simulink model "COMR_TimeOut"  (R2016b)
settings: Solver=FixedStepDiscrete  StartTime=0.0  StopTime=10.0  FixedStep=0.01  RelTol=1e-3  EnableMultiTasking=on
undefined symbols (not defined in the file or in its folder): bin2dec, COMR_cntObcTmtDiag_CW, COMR_cntVcu2A3TmtDiag_CW, COMR_flgTmtCAB_C, COMR_numPackVcuMsg_C, COMR_tiBusoffDiagEna_C, COMR_tiCabMsgTmt_C, COMR_tiCSCMsgTmt_C, COMR_tiGWMsg050Tmt_C, COMR_tiGWMsgTmt_C, COMR_tiHv638MsgTmt_C, COMR_tiMcuMsgTmt_C, COMR_tiObcMsgTmt_C, COMR_tiPackVcuMsgTmt_C, COMR_tiPwrupDiagEna_C, COMR_tiTmtBase_C, COMR_tiVcuMsgTmt_C, COMR_UAESFltDiagDisbl_C
libraries: simulink x167
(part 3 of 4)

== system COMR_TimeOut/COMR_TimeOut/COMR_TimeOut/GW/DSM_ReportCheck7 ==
  note: Fault report to diagnostic management system
  Dfc_id_nv : Inport  OutDataTypeStr=uint8
  Err : Inport  Port=2
  Heal : Inport  Port=3
  Bit Clear1 : simulink/Logic and Bit Operations/Bit Clear  iBit=4
  Bit Clear2 : simulink/Logic and Bit Operations/Bit Clear  iBit=3
  Bit Set : simulink/Logic and Bit Operations/Bit Set  iBit=4
  Bit Set1 : simulink/Logic and Bit Operations/Bit Set  iBit=3
  Bit Set2 : simulink/Logic and Bit Operations/Bit Set  iBit=3
  Bit Set4 : simulink/Logic and Bit Operations/Bit Set  iBit=7
  Constant1 : Constant  Value=0  OutDataTypeStr=uint8
  Constant7 : Constant  Value=0  OutDataTypeStr=boolean
  Delay2 : Delay  DelayLength=1  InitialCondition=1
  Delay3 : Delay  DelayLength=1  InitialCondition=0
  Logical Operator : Logic  Operator=OR  AllPortsSameDT=off  OutDataTypeStr=boolean
  Switch{1..4} (4 alike) : Switch  Criteria=u2 ~= 0
  Dfc_id : Outport  OutDataTypeStr=uint8
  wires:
  Switch1/1 -> Dfc_id/1
  Constant1/1 -> Switch1/3
  Logical Operator/1 -> Switch1/2
  Heal/1 -> Switch4/2, Logical Operator/1
  Delay3/1 -> Switch4/3
  Bit Clear1/1 -> Bit Set2/1
  Bit Set2/1 -> Switch4/1
  Err/1 -> Switch3/2, Logical Operator/2
  Switch4/1 -> Switch3/3
  Bit Set/1 -> Bit Set1/1
  Bit Set1/1 -> Switch3/1
  Switch2/1 -> Switch1/1, Delay3/1
  Bit Clear2/1 -> Switch2/1
  Switch3/1 -> Switch2/3
  Delay2/1 -> Switch2/2
  Constant7/1 -> Delay2/1
  Bit Set4/1 -> Bit Set/1
  Dfc_id_nv/1 -> Bit Clear1/1, Bit Set4/1, Bit Clear2/1

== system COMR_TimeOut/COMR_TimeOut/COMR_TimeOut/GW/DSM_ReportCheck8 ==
  note: Fault report to diagnostic management system
  Dfc_id_nv : Inport  OutDataTypeStr=uint8
  Err : Inport  Port=2
  Heal : Inport  Port=3
  Bit Clear1 : simulink/Logic and Bit Operations/Bit Clear  iBit=4
  Bit Clear2 : simulink/Logic and Bit Operations/Bit Clear  iBit=3
  Bit Set : simulink/Logic and Bit Operations/Bit Set  iBit=4
  Bit Set1 : simulink/Logic and Bit Operations/Bit Set  iBit=3
  Bit Set2 : simulink/Logic and Bit Operations/Bit Set  iBit=3
  Bit Set4 : simulink/Logic and Bit Operations/Bit Set  iBit=7
  Constant1 : Constant  Value=0  OutDataTypeStr=uint8
  Constant7 : Constant  Value=0  OutDataTypeStr=boolean
  Delay2 : Delay  DelayLength=1  InitialCondition=1
  Delay3 : Delay  DelayLength=1  InitialCondition=0
  Logical Operator : Logic  Operator=OR  AllPortsSameDT=off  OutDataTypeStr=boolean
  Switch{1..4} (4 alike) : Switch  Criteria=u2 ~= 0
  Dfc_id : Outport  OutDataTypeStr=uint8
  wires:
  Dfc_id_nv/1 -> Bit Clear2/1, Bit Set4/1, Bit Clear1/1
  Bit Set4/1 -> Bit Set/1
  Constant7/1 -> Delay2/1
  Delay2/1 -> Switch2/2
  Switch3/1 -> Switch2/3
  Bit Clear2/1 -> Switch2/1
  Switch2/1 -> Delay3/1, Switch1/1
  Bit Set1/1 -> Switch3/1
  Bit Set/1 -> Bit Set1/1
  Switch4/1 -> Switch3/3
  Err/1 -> Logical Operator/2, Switch3/2
  Bit Set2/1 -> Switch4/1
  Bit Clear1/1 -> Bit Set2/1
  Delay3/1 -> Switch4/3
  Heal/1 -> Logical Operator/1, Switch4/2
  Logical Operator/1 -> Switch1/2
  Constant1/1 -> Switch1/3
  Switch1/1 -> Dfc_id/1

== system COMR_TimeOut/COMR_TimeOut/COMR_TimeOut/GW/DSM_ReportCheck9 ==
  note: Fault report to diagnostic management system
  Dfc_id_nv : Inport  OutDataTypeStr=uint8
  Err : Inport  Port=2
  Heal : Inport  Port=3
  Bit Clear1 : simulink/Logic and Bit Operations/Bit Clear  iBit=4
  Bit Clear2 : simulink/Logic and Bit Operations/Bit Clear  iBit=3
  Bit Set : simulink/Logic and Bit Operations/Bit Set  iBit=4
  Bit Set1 : simulink/Logic and Bit Operations/Bit Set  iBit=3
  Bit Set2 : simulink/Logic and Bit Operations/Bit Set  iBit=3
  Bit Set4 : simulink/Logic and Bit Operations/Bit Set  iBit=7
  Constant1 : Constant  Value=0  OutDataTypeStr=uint8
  Constant7 : Constant  Value=0  OutDataTypeStr=boolean
  Delay2 : Delay  DelayLength=1  InitialCondition=1
  Delay3 : Delay  DelayLength=1  InitialCondition=0
  Logical Operator : Logic  Operator=OR  AllPortsSameDT=off  OutDataTypeStr=boolean
  Switch{1..4} (4 alike) : Switch  Criteria=u2 ~= 0
  Dfc_id : Outport  OutDataTypeStr=uint8
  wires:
  Switch1/1 -> Dfc_id/1
  Constant1/1 -> Switch1/3
  Logical Operator/1 -> Switch1/2
  Heal/1 -> Switch4/2, Logical Operator/1
  Delay3/1 -> Switch4/3
  Bit Clear1/1 -> Bit Set2/1
  Bit Set2/1 -> Switch4/1
  Err/1 -> Switch3/2, Logical Operator/2
  Switch4/1 -> Switch3/3
  Bit Set/1 -> Bit Set1/1
  Bit Set1/1 -> Switch3/1
  Switch2/1 -> Switch1/1, Delay3/1
  Bit Clear2/1 -> Switch2/1
  Switch3/1 -> Switch2/3
  Delay2/1 -> Switch2/2
  Constant7/1 -> Delay2/1
  Bit Set4/1 -> Bit Set/1
  Dfc_id_nv/1 -> Bit Clear1/1, Bit Set4/1, Bit Clear2/1

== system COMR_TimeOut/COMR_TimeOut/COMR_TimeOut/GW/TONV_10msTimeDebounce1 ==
  note: Turn On Delay Time Deboune
  u : Inport
  T : Inport  Port=2
  Add : Sum
  Constant1 : Constant  Value=0  OutDataTypeStr=single
  Constant2 : Constant  OutDataTypeStr=uint8
  Constant3 : Constant  Value=0  OutDataTypeStr=uint8
  Constant4 : Constant  Value=0.01  OutDataTypeStr=single
  Delay : Delay  DelayLength=1  InitialCondition=0
  MinMax : MinMax  Inputs=2
  Product : Product  OutMin=[0]  OutMax=[65535]  OutDataTypeStr=single
  Relational Operator : RelationalOperator  Operator=>  OutDataTypeStr=boolean  RndMeth=Simplest
  Switch : Switch  Criteria=u2 ~= 0
  Switch1 : Switch  Criteria=u2 ~= 0
  y : Outport
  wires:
  Switch1/1 -> Product/1
  Constant3/1 -> Switch1/3
  Constant2/1 -> Switch1/1
  u/1 -> Switch1/2, Switch/2
  Constant4/1 -> Switch/1
  Constant1/1 -> Switch/3
  Add/1 -> Product/2
  Product/1 -> Relational Operator/1, Delay/1
  Switch/1 -> Add/1
  Delay/1 -> MinMax/2
  Relational Operator/1 -> y/1
  T/1 -> MinMax/1, Relational Operator/2
  MinMax/1 -> Add/2

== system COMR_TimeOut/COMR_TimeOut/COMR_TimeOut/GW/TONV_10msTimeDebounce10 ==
  note: Turn On Delay Time Deboune
  u : Inport
  T : Inport  Port=2
  Add : Sum
  Constant1 : Constant  Value=0  OutDataTypeStr=single
  Constant2 : Constant  OutDataTypeStr=uint8
  Constant3 : Constant  Value=0  OutDataTypeStr=uint8
  Constant4 : Constant  Value=0.01  OutDataTypeStr=single
  Delay : Delay  DelayLength=1  InitialCondition=0
  MinMax : MinMax  Inputs=2
  Product : Product  OutMin=[0]  OutMax=[65535]  OutDataTypeStr=single
  Relational Operator : RelationalOperator  Operator=>  OutDataTypeStr=boolean  RndMeth=Simplest
  Switch : Switch  Criteria=u2 ~= 0
  Switch1 : Switch  Criteria=u2 ~= 0
  y : Outport
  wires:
  Switch1/1 -> Product/1
  Constant3/1 -> Switch1/3
  Constant2/1 -> Switch1/1
  u/1 -> Switch1/2, Switch/2
  Constant4/1 -> Switch/1
  Constant1/1 -> Switch/3
  Add/1 -> Product/2
  Product/1 -> Relational Operator/1, Delay/1
  Switch/1 -> Add/1
  Delay/1 -> MinMax/2
  Relational Operator/1 -> y/1
  T/1 -> MinMax/1, Relational Operator/2
  MinMax/1 -> Add/2

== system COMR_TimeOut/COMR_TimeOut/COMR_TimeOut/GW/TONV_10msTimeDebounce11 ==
  note: Turn On Delay Time Deboune
  u : Inport
  T : Inport  Port=2
  Add : Sum
  Constant1 : Constant  Value=0  OutDataTypeStr=single
  Constant2 : Constant  OutDataTypeStr=uint8
  Constant3 : Constant  Value=0  OutDataTypeStr=uint8
  Constant4 : Constant  Value=0.01  OutDataTypeStr=single
  Delay : Delay  DelayLength=1  InitialCondition=0
  MinMax : MinMax  Inputs=2
  Product : Product  OutMin=[0]  OutMax=[65535]  OutDataTypeStr=single
  Relational Operator : RelationalOperator  Operator=>  OutDataTypeStr=boolean  RndMeth=Simplest
  Switch : Switch  Criteria=u2 ~= 0
  Switch1 : Switch  Criteria=u2 ~= 0
  y : Outport
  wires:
  Switch1/1 -> Product/1
  Constant3/1 -> Switch1/3
  Constant2/1 -> Switch1/1
  u/1 -> Switch1/2, Switch/2
  Constant4/1 -> Switch/1
  Constant1/1 -> Switch/3
  Add/1 -> Product/2
  Product/1 -> Relational Operator/1, Delay/1
  Switch/1 -> Add/1
  Delay/1 -> MinMax/2
  Relational Operator/1 -> y/1
  T/1 -> MinMax/1, Relational Operator/2
  MinMax/1 -> Add/2

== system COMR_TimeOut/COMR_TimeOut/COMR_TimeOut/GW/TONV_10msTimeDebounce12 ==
  note: Turn On Delay Time Deboune
  u : Inport
  T : Inport  Port=2
  Add : Sum
  Constant1 : Constant  Value=0  OutDataTypeStr=single
  Constant2 : Constant  OutDataTypeStr=uint8
  Constant3 : Constant  Value=0  OutDataTypeStr=uint8
  Constant4 : Constant  Value=0.01  OutDataTypeStr=single
  Delay : Delay  DelayLength=1  InitialCondition=0
  MinMax : MinMax  Inputs=2
  Product : Product  OutMin=[0]  OutMax=[65535]  OutDataTypeStr=single
  Relational Operator : RelationalOperator  Operator=>  OutDataTypeStr=boolean  RndMeth=Simplest
  Switch : Switch  Criteria=u2 ~= 0
  Switch1 : Switch  Criteria=u2 ~= 0
  y : Outport
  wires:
  Switch1/1 -> Product/1
  Constant3/1 -> Switch1/3
  Constant2/1 -> Switch1/1
  u/1 -> Switch1/2, Switch/2
  Constant4/1 -> Switch/1
  Constant1/1 -> Switch/3
  Add/1 -> Product/2
  Product/1 -> Relational Operator/1, Delay/1
  Switch/1 -> Add/1
  Delay/1 -> MinMax/2
  Relational Operator/1 -> y/1
  T/1 -> MinMax/1, Relational Operator/2
  MinMax/1 -> Add/2

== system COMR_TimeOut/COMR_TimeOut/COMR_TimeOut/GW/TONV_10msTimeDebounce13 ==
  note: Turn On Delay Time Deboune
  u : Inport
  T : Inport  Port=2
  Add : Sum
  Constant1 : Constant  Value=0  OutDataTypeStr=single
  Constant2 : Constant  OutDataTypeStr=uint8
  Constant3 : Constant  Value=0  OutDataTypeStr=uint8
  Constant4 : Constant  Value=0.01  OutDataTypeStr=single
  Delay : Delay  DelayLength=1  InitialCondition=0
  MinMax : MinMax  Inputs=2
  Product : Product  OutMin=[0]  OutMax=[65535]  OutDataTypeStr=single
  Relational Operator : RelationalOperator  Operator=>  OutDataTypeStr=boolean  RndMeth=Simplest
  Switch : Switch  Criteria=u2 ~= 0
  Switch1 : Switch  Criteria=u2 ~= 0
  y : Outport
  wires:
  Switch1/1 -> Product/1
  Constant3/1 -> Switch1/3
  Constant2/1 -> Switch1/1
  u/1 -> Switch1/2, Switch/2
  Constant4/1 -> Switch/1
  Constant1/1 -> Switch/3
  Add/1 -> Product/2
  Product/1 -> Relational Operator/1, Delay/1
  Switch/1 -> Add/1
  Delay/1 -> MinMax/2
  Relational Operator/1 -> y/1
  T/1 -> MinMax/1, Relational Operator/2
  MinMax/1 -> Add/2

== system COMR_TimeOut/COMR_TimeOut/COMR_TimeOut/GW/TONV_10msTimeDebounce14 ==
  note: Turn On Delay Time Deboune
  u : Inport
  T : Inport  Port=2
  Add : Sum
  Constant1 : Constant  Value=0  OutDataTypeStr=single
  Constant2 : Constant  OutDataTypeStr=uint8
  Constant3 : Constant  Value=0  OutDataTypeStr=uint8
  Constant4 : Constant  Value=0.01  OutDataTypeStr=single
  Delay : Delay  DelayLength=1  InitialCondition=0
  MinMax : MinMax  Inputs=2
  Product : Product  OutMin=[0]  OutMax=[65535]  OutDataTypeStr=single
  Relational Operator : RelationalOperator  Operator=>  OutDataTypeStr=boolean  RndMeth=Simplest
  Switch : Switch  Criteria=u2 ~= 0
  Switch1 : Switch  Criteria=u2 ~= 0
  y : Outport
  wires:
  Switch1/1 -> Product/1
  Constant3/1 -> Switch1/3
  Constant2/1 -> Switch1/1
  u/1 -> Switch1/2, Switch/2
  Constant4/1 -> Switch/1
  Constant1/1 -> Switch/3
  Add/1 -> Product/2
  Product/1 -> Relational Operator/1, Delay/1
  Switch/1 -> Add/1
  Delay/1 -> MinMax/2
  Relational Operator/1 -> y/1
  T/1 -> MinMax/1, Relational Operator/2
  MinMax/1 -> Add/2

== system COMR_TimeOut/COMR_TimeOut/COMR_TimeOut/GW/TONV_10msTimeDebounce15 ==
  note: Turn On Delay Time Deboune
  u : Inport
  T : Inport  Port=2
  Add : Sum
  Constant1 : Constant  Value=0  OutDataTypeStr=single
  Constant2 : Constant  OutDataTypeStr=uint8
  Constant3 : Constant  Value=0  OutDataTypeStr=uint8
  Constant4 : Constant  Value=0.01  OutDataTypeStr=single
  Delay : Delay  DelayLength=1  InitialCondition=0
  MinMax : MinMax  Inputs=2
  Product : Product  OutMin=[0]  OutMax=[65535]  OutDataTypeStr=single
  Relational Operator : RelationalOperator  Operator=>  OutDataTypeStr=boolean  RndMeth=Simplest
  Switch : Switch  Criteria=u2 ~= 0
  Switch1 : Switch  Criteria=u2 ~= 0
  y : Outport
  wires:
  Switch1/1 -> Product/1
  Constant3/1 -> Switch1/3
  Constant2/1 -> Switch1/1
  u/1 -> Switch1/2, Switch/2
  Constant4/1 -> Switch/1
  Constant1/1 -> Switch/3
  Add/1 -> Product/2
  Product/1 -> Relational Operator/1, Delay/1
  Switch/1 -> Add/1
  Delay/1 -> MinMax/2
  Relational Operator/1 -> y/1
  T/1 -> MinMax/1, Relational Operator/2
  MinMax/1 -> Add/2

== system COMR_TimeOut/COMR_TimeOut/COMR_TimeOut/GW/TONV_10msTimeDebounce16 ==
  note: Turn On Delay Time Deboune
  u : Inport
  T : Inport  Port=2
  Add : Sum
  Constant1 : Constant  Value=0  OutDataTypeStr=single
  Constant2 : Constant  OutDataTypeStr=uint8
  Constant3 : Constant  Value=0  OutDataTypeStr=uint8
  Constant4 : Constant  Value=0.01  OutDataTypeStr=single
  Delay : Delay  DelayLength=1  InitialCondition=0
  MinMax : MinMax  Inputs=2
  Product : Product  OutMin=[0]  OutMax=[65535]  OutDataTypeStr=single
  Relational Operator : RelationalOperator  Operator=>  OutDataTypeStr=boolean  RndMeth=Simplest
  Switch : Switch  Criteria=u2 ~= 0
  Switch1 : Switch  Criteria=u2 ~= 0
  y : Outport
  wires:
  Switch1/1 -> Product/1
  Constant3/1 -> Switch1/3
  Constant2/1 -> Switch1/1
  u/1 -> Switch1/2, Switch/2
  Constant4/1 -> Switch/1
  Constant1/1 -> Switch/3
  Add/1 -> Product/2
  Product/1 -> Relational Operator/1, Delay/1
  Switch/1 -> Add/1
  Delay/1 -> MinMax/2
  Relational Operator/1 -> y/1
  T/1 -> MinMax/1, Relational Operator/2
  MinMax/1 -> Add/2

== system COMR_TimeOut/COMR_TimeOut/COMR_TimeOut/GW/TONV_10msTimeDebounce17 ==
  note: Turn On Delay Time Deboune
  u : Inport
  T : Inport  Port=2
  Add : Sum
  Constant1 : Constant  Value=0  OutDataTypeStr=single
  Constant2 : Constant  OutDataTypeStr=uint8
  Constant3 : Constant  Value=0  OutDataTypeStr=uint8
  Constant4 : Constant  Value=0.01  OutDataTypeStr=single
  Delay : Delay  DelayLength=1  InitialCondition=0
  MinMax : MinMax  Inputs=2
  Product : Product  OutMin=[0]  OutMax=[65535]  OutDataTypeStr=single
  Relational Operator : RelationalOperator  Operator=>  OutDataTypeStr=boolean  RndMeth=Simplest
  Switch : Switch  Criteria=u2 ~= 0
  Switch1 : Switch  Criteria=u2 ~= 0
  y : Outport
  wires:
  Switch1/1 -> Product/1
  Constant3/1 -> Switch1/3
  Constant2/1 -> Switch1/1
  u/1 -> Switch1/2, Switch/2
  Constant4/1 -> Switch/1
  Constant1/1 -> Switch/3
  Add/1 -> Product/2
  Product/1 -> Relational Operator/1, Delay/1
  Switch/1 -> Add/1
  Delay/1 -> MinMax/2
  Relational Operator/1 -> y/1
  T/1 -> MinMax/1, Relational Operator/2
  MinMax/1 -> Add/2

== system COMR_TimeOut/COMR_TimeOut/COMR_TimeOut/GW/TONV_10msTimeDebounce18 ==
  note: Turn On Delay Time Deboune
  u : Inport
  T : Inport  Port=2
  Add : Sum
  Constant1 : Constant  Value=0  OutDataTypeStr=single
  Constant2 : Constant  OutDataTypeStr=uint8
  Constant3 : Constant  Value=0  OutDataTypeStr=uint8
  Constant4 : Constant  Value=0.01  OutDataTypeStr=single
  Delay : Delay  DelayLength=1  InitialCondition=0
  MinMax : MinMax  Inputs=2
  Product : Product  OutMin=[0]  OutMax=[65535]  OutDataTypeStr=single
  Relational Operator : RelationalOperator  Operator=>  OutDataTypeStr=boolean  RndMeth=Simplest
  Switch : Switch  Criteria=u2 ~= 0
  Switch1 : Switch  Criteria=u2 ~= 0
  y : Outport
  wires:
  Switch1/1 -> Product/1
  Constant3/1 -> Switch1/3
  Constant2/1 -> Switch1/1
  u/1 -> Switch1/2, Switch/2
  Constant4/1 -> Switch/1
  Constant1/1 -> Switch/3
  Add/1 -> Product/2
  Product/1 -> Relational Operator/1, Delay/1
  Switch/1 -> Add/1
  Delay/1 -> MinMax/2
  Relational Operator/1 -> y/1
  T/1 -> MinMax/1, Relational Operator/2
  MinMax/1 -> Add/2

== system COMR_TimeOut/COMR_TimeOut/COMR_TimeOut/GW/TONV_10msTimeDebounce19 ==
  note: Turn On Delay Time Deboune
  u : Inport
  T : Inport  Port=2
  Add : Sum
  Constant1 : Constant  Value=0  OutDataTypeStr=single
  Constant2 : Constant  OutDataTypeStr=uint8
  Constant3 : Constant  Value=0  OutDataTypeStr=uint8
  Constant4 : Constant  Value=0.01  OutDataTypeStr=single
  Delay : Delay  DelayLength=1  InitialCondition=0
  MinMax : MinMax  Inputs=2
  Product : Product  OutMin=[0]  OutMax=[65535]  OutDataTypeStr=single
  Relational Operator : RelationalOperator  Operator=>  OutDataTypeStr=boolean  RndMeth=Simplest
  Switch : Switch  Criteria=u2 ~= 0
  Switch1 : Switch  Criteria=u2 ~= 0
  y : Outport
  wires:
  Switch1/1 -> Product/1
  Constant3/1 -> Switch1/3
  Constant2/1 -> Switch1/1
  u/1 -> Switch1/2, Switch/2
  Constant4/1 -> Switch/1
  Constant1/1 -> Switch/3
  Add/1 -> Product/2
  Product/1 -> Relational Operator/1, Delay/1
  Switch/1 -> Add/1
  Delay/1 -> MinMax/2
  Relational Operator/1 -> y/1
  T/1 -> MinMax/1, Relational Operator/2
  MinMax/1 -> Add/2

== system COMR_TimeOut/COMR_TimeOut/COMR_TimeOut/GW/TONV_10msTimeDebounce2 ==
  note: Turn On Delay Time Deboune
  u : Inport
  T : Inport  Port=2
  Add : Sum
  Constant1 : Constant  Value=0  OutDataTypeStr=single
  Constant2 : Constant  OutDataTypeStr=uint8
  Constant3 : Constant  Value=0  OutDataTypeStr=uint8
  Constant4 : Constant  Value=0.01  OutDataTypeStr=single
  Delay : Delay  DelayLength=1  InitialCondition=0
  MinMax : MinMax  Inputs=2
  Product : Product  OutMin=[0]  OutMax=[65535]  OutDataTypeStr=single
  Relational Operator : RelationalOperator  Operator=>  OutDataTypeStr=boolean  RndMeth=Simplest
  Switch : Switch  Criteria=u2 ~= 0
  Switch1 : Switch  Criteria=u2 ~= 0
  y : Outport
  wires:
  Switch1/1 -> Product/1
  Constant3/1 -> Switch1/3
  Constant2/1 -> Switch1/1
  u/1 -> Switch1/2, Switch/2
  Constant4/1 -> Switch/1
  Constant1/1 -> Switch/3
  Add/1 -> Product/2
  Product/1 -> Relational Operator/1, Delay/1
  Switch/1 -> Add/1
  Delay/1 -> MinMax/2
  Relational Operator/1 -> y/1
  T/1 -> MinMax/1, Relational Operator/2
  MinMax/1 -> Add/2

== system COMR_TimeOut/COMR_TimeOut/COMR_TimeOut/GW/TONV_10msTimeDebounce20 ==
  note: Turn On Delay Time Deboune
  u : Inport
  T : Inport  Port=2
  Add : Sum
  Constant1 : Constant  Value=0  OutDataTypeStr=single
  Constant2 : Constant  OutDataTypeStr=uint8
  Constant3 : Constant  Value=0  OutDataTypeStr=uint8
  Constant4 : Constant  Value=0.01  OutDataTypeStr=single
  Delay : Delay  DelayLength=1  InitialCondition=0
  MinMax : MinMax  Inputs=2
  Product : Product  OutMin=[0]  OutMax=[65535]  OutDataTypeStr=single
  Relational Operator : RelationalOperator  Operator=>  OutDataTypeStr=boolean  RndMeth=Simplest
  Switch : Switch  Criteria=u2 ~= 0
  Switch1 : Switch  Criteria=u2 ~= 0
  y : Outport
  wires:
  Switch1/1 -> Product/1
  Constant3/1 -> Switch1/3
  Constant2/1 -> Switch1/1
  u/1 -> Switch1/2, Switch/2
  Constant4/1 -> Switch/1
  Constant1/1 -> Switch/3
  Add/1 -> Product/2
  Product/1 -> Relational Operator/1, Delay/1
  Switch/1 -> Add/1
  Delay/1 -> MinMax/2
  Relational Operator/1 -> y/1
  T/1 -> MinMax/1, Relational Operator/2
  MinMax/1 -> Add/2

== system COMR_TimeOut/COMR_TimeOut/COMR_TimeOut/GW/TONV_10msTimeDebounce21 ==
  note: Turn On Delay Time Deboune
  u : Inport
  T : Inport  Port=2
  Add : Sum
  Constant1 : Constant  Value=0  OutDataTypeStr=single
  Constant2 : Constant  OutDataTypeStr=uint8
  Constant3 : Constant  Value=0  OutDataTypeStr=uint8
  Constant4 : Constant  Value=0.01  OutDataTypeStr=single
  Delay : Delay  DelayLength=1  InitialCondition=0
  MinMax : MinMax  Inputs=2
  Product : Product  OutMin=[0]  OutMax=[65535]  OutDataTypeStr=single
  Relational Operator : RelationalOperator  Operator=>  OutDataTypeStr=boolean  RndMeth=Simplest
  Switch : Switch  Criteria=u2 ~= 0
  Switch1 : Switch  Criteria=u2 ~= 0
  y : Outport
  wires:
  Switch1/1 -> Product/1
  Constant3/1 -> Switch1/3
  Constant2/1 -> Switch1/1
  u/1 -> Switch1/2, Switch/2
  Constant4/1 -> Switch/1
  Constant1/1 -> Switch/3
  Add/1 -> Product/2
  Product/1 -> Relational Operator/1, Delay/1
  Switch/1 -> Add/1
  Delay/1 -> MinMax/2
  Relational Operator/1 -> y/1
  T/1 -> MinMax/1, Relational Operator/2
  MinMax/1 -> Add/2

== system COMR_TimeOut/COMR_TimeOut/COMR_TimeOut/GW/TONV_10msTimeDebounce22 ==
  note: Turn On Delay Time Deboune
  u : Inport
  T : Inport  Port=2
  Add : Sum
  Constant1 : Constant  Value=0  OutDataTypeStr=single
  Constant2 : Constant  OutDataTypeStr=uint8
  Constant3 : Constant  Value=0  OutDataTypeStr=uint8
  Constant4 : Constant  Value=0.01  OutDataTypeStr=single
  Delay : Delay  DelayLength=1  InitialCondition=0
  MinMax : MinMax  Inputs=2
  Product : Product  OutMin=[0]  OutMax=[65535]  OutDataTypeStr=single
  Relational Operator : RelationalOperator  Operator=>  OutDataTypeStr=boolean  RndMeth=Simplest
  Switch : Switch  Criteria=u2 ~= 0
  Switch1 : Switch  Criteria=u2 ~= 0
  y : Outport
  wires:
  Switch1/1 -> Product/1
  Constant3/1 -> Switch1/3
  Constant2/1 -> Switch1/1
  u/1 -> Switch1/2, Switch/2
  Constant4/1 -> Switch/1
  Constant1/1 -> Switch/3
  Add/1 -> Product/2
  Product/1 -> Relational Operator/1, Delay/1
  Switch/1 -> Add/1
  Delay/1 -> MinMax/2
  Relational Operator/1 -> y/1
  T/1 -> MinMax/1, Relational Operator/2
  MinMax/1 -> Add/2

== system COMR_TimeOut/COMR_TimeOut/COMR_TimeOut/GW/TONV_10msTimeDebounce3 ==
  note: Turn On Delay Time Deboune
  u : Inport
  T : Inport  Port=2
  Add : Sum
  Constant1 : Constant  Value=0  OutDataTypeStr=single
  Constant2 : Constant  OutDataTypeStr=uint8
  Constant3 : Constant  Value=0  OutDataTypeStr=uint8
  Constant4 : Constant  Value=0.01  OutDataTypeStr=single
  Delay : Delay  DelayLength=1  InitialCondition=0
  MinMax : MinMax  Inputs=2
  Product : Product  OutMin=[0]  OutMax=[65535]  OutDataTypeStr=single
  Relational Operator : RelationalOperator  Operator=>  OutDataTypeStr=boolean  RndMeth=Simplest
  Switch : Switch  Criteria=u2 ~= 0
  Switch1 : Switch  Criteria=u2 ~= 0
  y : Outport
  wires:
  Switch1/1 -> Product/1
  Constant3/1 -> Switch1/3
  Constant2/1 -> Switch1/1
  u/1 -> Switch1/2, Switch/2
  Constant4/1 -> Switch/1
  Constant1/1 -> Switch/3
  Add/1 -> Product/2
  Product/1 -> Relational Operator/1, Delay/1
  Switch/1 -> Add/1
  Delay/1 -> MinMax/2
  Relational Operator/1 -> y/1
  T/1 -> MinMax/1, Relational Operator/2
  MinMax/1 -> Add/2

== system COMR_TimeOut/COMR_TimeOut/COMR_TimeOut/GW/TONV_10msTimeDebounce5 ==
  note: Turn On Delay Time Deboune
  u : Inport
  T : Inport  Port=2
  Add : Sum
  Constant1 : Constant  Value=0  OutDataTypeStr=single
  Constant2 : Constant  OutDataTypeStr=uint8
  Constant3 : Constant  Value=0  OutDataTypeStr=uint8
  Constant4 : Constant  Value=0.01  OutDataTypeStr=single
  Delay : Delay  DelayLength=1  InitialCondition=0
  MinMax : MinMax  Inputs=2
  Product : Product  OutMin=[0]  OutMax=[65535]  OutDataTypeStr=single
  Relational Operator : RelationalOperator  Operator=>  OutDataTypeStr=boolean  RndMeth=Simplest
  Switch : Switch  Criteria=u2 ~= 0
  Switch1 : Switch  Criteria=u2 ~= 0
  y : Outport
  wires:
  Switch1/1 -> Product/1
  Constant3/1 -> Switch1/3
  Constant2/1 -> Switch1/1
  u/1 -> Switch1/2, Switch/2
  Constant4/1 -> Switch/1
  Constant1/1 -> Switch/3
  Add/1 -> Product/2
  Product/1 -> Relational Operator/1, Delay/1
  Switch/1 -> Add/1
  Delay/1 -> MinMax/2
  Relational Operator/1 -> y/1
  T/1 -> MinMax/1, Relational Operator/2
  MinMax/1 -> Add/2

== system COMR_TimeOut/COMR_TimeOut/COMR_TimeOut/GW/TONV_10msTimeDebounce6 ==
  note: Turn On Delay Time Deboune
  u : Inport
  T : Inport  Port=2
  Add : Sum
  Constant1 : Constant  Value=0  OutDataTypeStr=single
  Constant2 : Constant  OutDataTypeStr=uint8
  Constant3 : Constant  Value=0  OutDataTypeStr=uint8
  Constant4 : Constant  Value=0.01  OutDataTypeStr=single
  Delay : Delay  DelayLength=1  InitialCondition=0
  MinMax : MinMax  Inputs=2
  Product : Product  OutMin=[0]  OutMax=[65535]  OutDataTypeStr=single
  Relational Operator : RelationalOperator  Operator=>  OutDataTypeStr=boolean  RndMeth=Simplest
  Switch : Switch  Criteria=u2 ~= 0
  Switch1 : Switch  Criteria=u2 ~= 0
  y : Outport
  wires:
  Switch1/1 -> Product/1
  Constant3/1 -> Switch1/3
  Constant2/1 -> Switch1/1
  u/1 -> Switch1/2, Switch/2
  Constant4/1 -> Switch/1
  Constant1/1 -> Switch/3
  Add/1 -> Product/2
  Product/1 -> Relational Operator/1, Delay/1
  Switch/1 -> Add/1
  Delay/1 -> MinMax/2
  Relational Operator/1 -> y/1
  T/1 -> MinMax/1, Relational Operator/2
  MinMax/1 -> Add/2

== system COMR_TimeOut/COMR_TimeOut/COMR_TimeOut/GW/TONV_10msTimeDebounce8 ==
  note: Turn On Delay Time Deboune
  u : Inport
  T : Inport  Port=2
  Add : Sum
  Constant1 : Constant  Value=0  OutDataTypeStr=single
  Constant2 : Constant  OutDataTypeStr=uint8
  Constant3 : Constant  Value=0  OutDataTypeStr=uint8
  Constant4 : Constant  Value=0.01  OutDataTypeStr=single
  Delay : Delay  DelayLength=1  InitialCondition=0
  MinMax : MinMax  Inputs=2
  Product : Product  OutMin=[0]  OutMax=[65535]  OutDataTypeStr=single
  Relational Operator : RelationalOperator  Operator=>  OutDataTypeStr=boolean  RndMeth=Simplest
  Switch : Switch  Criteria=u2 ~= 0
  Switch1 : Switch  Criteria=u2 ~= 0
  y : Outport
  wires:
  Switch1/1 -> Product/1
  Constant3/1 -> Switch1/3
  Constant2/1 -> Switch1/1
  u/1 -> Switch1/2, Switch/2
  Constant4/1 -> Switch/1
  Constant1/1 -> Switch/3
  Add/1 -> Product/2
  Product/1 -> Relational Operator/1, Delay/1
  Switch/1 -> Add/1
  Delay/1 -> MinMax/2
  Relational Operator/1 -> y/1
  T/1 -> MinMax/1, Relational Operator/2
  MinMax/1 -> Add/2

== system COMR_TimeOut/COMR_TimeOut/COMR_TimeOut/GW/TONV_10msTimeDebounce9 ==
  note: Turn On Delay Time Deboune
  u : Inport
  T : Inport  Port=2
  Add : Sum
  Constant1 : Constant  Value=0  OutDataTypeStr=single
  Constant2 : Constant  OutDataTypeStr=uint8
  Constant3 : Constant  Value=0  OutDataTypeStr=uint8
  Constant4 : Constant  Value=0.01  OutDataTypeStr=single
  Delay : Delay  DelayLength=1  InitialCondition=0
  MinMax : MinMax  Inputs=2
  Product : Product  OutMin=[0]  OutMax=[65535]  OutDataTypeStr=single
  Relational Operator : RelationalOperator  Operator=>  OutDataTypeStr=boolean  RndMeth=Simplest
  Switch : Switch  Criteria=u2 ~= 0
  Switch1 : Switch  Criteria=u2 ~= 0
  y : Outport
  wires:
  Switch1/1 -> Product/1
  Constant3/1 -> Switch1/3
  Constant2/1 -> Switch1/1
  u/1 -> Switch1/2, Switch/2
  Constant4/1 -> Switch/1
  Constant1/1 -> Switch/3
  Add/1 -> Product/2
  Product/1 -> Relational Operator/1, Delay/1
  Switch/1 -> Add/1
  Delay/1 -> MinMax/2
  Relational Operator/1 -> y/1
  T/1 -> MinMax/1, Relational Operator/2
  MinMax/1 -> Add/2

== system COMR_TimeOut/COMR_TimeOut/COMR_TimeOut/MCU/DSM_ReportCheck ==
  note: Fault report to diagnostic management system
  Dfc_id_nv : Inport  OutDataTypeStr=uint8
  Err : Inport  Port=2
  Heal : Inport  Port=3
  Bit Clear1 : simulink/Logic and Bit Operations/Bit Clear  iBit=4
  Bit Clear2 : simulink/Logic and Bit Operations/Bit Clear  iBit=3
  Bit Set : simulink/Logic and Bit Operations/Bit Set  iBit=4
  Bit Set1 : simulink/Logic and Bit Operations/Bit Set  iBit=3
  Bit Set2 : simulink/Logic and Bit Operations/Bit Set  iBit=3
  Bit Set4 : simulink/Logic and Bit Operations/Bit Set  iBit=7
  Constant1 : Constant  Value=0  OutDataTypeStr=uint8
  Constant7 : Constant  Value=0  OutDataTypeStr=boolean
  Delay2 : Delay  DelayLength=1  InitialCondition=1
  Delay3 : Delay  DelayLength=1  InitialCondition=0
  Logical Operator : Logic  Operator=OR  AllPortsSameDT=off  OutDataTypeStr=boolean
  Switch{1..4} (4 alike) : Switch  Criteria=u2 ~= 0
  Dfc_id : Outport  OutDataTypeStr=uint8
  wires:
  Dfc_id_nv/1 -> Bit Clear2/1, Bit Set4/1, Bit Clear1/1
  Bit Set4/1 -> Bit Set/1
  Constant7/1 -> Delay2/1
  Delay2/1 -> Switch2/2
  Switch3/1 -> Switch2/3
  Bit Clear2/1 -> Switch2/1
  Switch2/1 -> Delay3/1, Switch1/1
  Bit Set1/1 -> Switch3/1
  Bit Set/1 -> Bit Set1/1
  Switch4/1 -> Switch3/3
  Err/1 -> Logical Operator/2, Switch3/2
  Bit Set2/1 -> Switch4/1
  Bit Clear1/1 -> Bit Set2/1
  Delay3/1 -> Switch4/3
  Heal/1 -> Logical Operator/1, Switch4/2
  Logical Operator/1 -> Switch1/2
  Constant1/1 -> Switch1/3
  Switch1/1 -> Dfc_id/1

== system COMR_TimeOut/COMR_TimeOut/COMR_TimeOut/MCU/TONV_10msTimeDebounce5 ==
  note: Turn On Delay Time Deboune
  u : Inport
  T : Inport  Port=2
  Add : Sum
  Constant1 : Constant  Value=0  OutDataTypeStr=single
  Constant2 : Constant  OutDataTypeStr=uint8
  Constant3 : Constant  Value=0  OutDataTypeStr=uint8
  Constant4 : Constant  Value=0.01  OutDataTypeStr=single
  Delay : Delay  DelayLength=1  InitialCondition=0
  MinMax : MinMax  Inputs=2
  Product : Product  OutMin=[0]  OutMax=[65535]  OutDataTypeStr=single
  Relational Operator : RelationalOperator  Operator=>  OutDataTypeStr=boolean  RndMeth=Simplest
  Switch : Switch  Criteria=u2 ~= 0
  Switch1 : Switch  Criteria=u2 ~= 0
  y : Outport
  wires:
  Switch1/1 -> Product/1
  Constant3/1 -> Switch1/3
  Constant2/1 -> Switch1/1
  u/1 -> Switch1/2, Switch/2
  Constant4/1 -> Switch/1
  Constant1/1 -> Switch/3
  Add/1 -> Product/2
  Product/1 -> Relational Operator/1, Delay/1
  Switch/1 -> Add/1
  Delay/1 -> MinMax/2
  Relational Operator/1 -> y/1
  T/1 -> MinMax/1, Relational Operator/2
  MinMax/1 -> Add/2

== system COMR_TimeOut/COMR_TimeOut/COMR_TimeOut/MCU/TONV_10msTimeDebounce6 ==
  note: Turn On Delay Time Deboune
  u : Inport
  T : Inport  Port=2
  Add : Sum
  Constant1 : Constant  Value=0  OutDataTypeStr=single
  Constant2 : Constant  OutDataTypeStr=uint8
  Constant3 : Constant  Value=0  OutDataTypeStr=uint8
  Constant4 : Constant  Value=0.01  OutDataTypeStr=single
  Delay : Delay  DelayLength=1  InitialCondition=0
  MinMax : MinMax  Inputs=2
  Product : Product  OutMin=[0]  OutMax=[65535]  OutDataTypeStr=single
  Relational Operator : RelationalOperator  Operator=>  OutDataTypeStr=boolean  RndMeth=Simplest
  Switch : Switch  Criteria=u2 ~= 0
  Switch1 : Switch  Criteria=u2 ~= 0
  y : Outport
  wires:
  Switch1/1 -> Product/1
  Constant3/1 -> Switch1/3
  Constant2/1 -> Switch1/1
  u/1 -> Switch1/2, Switch/2
  Constant4/1 -> Switch/1
  Constant1/1 -> Switch/3
  Add/1 -> Product/2
  Product/1 -> Relational Operator/1, Delay/1
  Switch/1 -> Add/1
  Delay/1 -> MinMax/2
  Relational Operator/1 -> y/1
  T/1 -> MinMax/1, Relational Operator/2
  MinMax/1 -> Add/2

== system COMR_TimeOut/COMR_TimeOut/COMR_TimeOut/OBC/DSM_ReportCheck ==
  note: Fault report to diagnostic management system
  Dfc_id_nv : Inport  OutDataTypeStr=uint8
  Err : Inport  Port=2
  Heal : Inport  Port=3
  Bit Clear1 : simulink/Logic and Bit Operations/Bit Clear  iBit=4
  Bit Clear2 : simulink/Logic and Bit Operations/Bit Clear  iBit=3
  Bit Set : simulink/Logic and Bit Operations/Bit Set  iBit=4
  Bit Set1 : simulink/Logic and Bit Operations/Bit Set  iBit=3
  Bit Set2 : simulink/Logic and Bit Operations/Bit Set  iBit=3
  Bit Set4 : simulink/Logic and Bit Operations/Bit Set  iBit=7
  Constant1 : Constant  Value=0  OutDataTypeStr=uint8
  Constant7 : Constant  Value=0  OutDataTypeStr=boolean
  Delay2 : Delay  DelayLength=1  InitialCondition=1
  Delay3 : Delay  DelayLength=1  InitialCondition=0
  Logical Operator : Logic  Operator=OR  AllPortsSameDT=off  OutDataTypeStr=boolean
  Switch{1..4} (4 alike) : Switch  Criteria=u2 ~= 0
  Dfc_id : Outport  OutDataTypeStr=uint8
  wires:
  Dfc_id_nv/1 -> Bit Clear2/1, Bit Set4/1, Bit Clear1/1
  Bit Set4/1 -> Bit Set/1
  Constant7/1 -> Delay2/1
  Delay2/1 -> Switch2/2
  Switch3/1 -> Switch2/3
  Bit Clear2/1 -> Switch2/1
  Switch2/1 -> Delay3/1, Switch1/1
  Bit Set1/1 -> Switch3/1
  Bit Set/1 -> Bit Set1/1
  Switch4/1 -> Switch3/3
  Err/1 -> Logical Operator/2, Switch3/2
  Bit Set2/1 -> Switch4/1
  Bit Clear1/1 -> Bit Set2/1
  Delay3/1 -> Switch4/3
  Heal/1 -> Logical Operator/1, Switch4/2
  Logical Operator/1 -> Switch1/2
  Constant1/1 -> Switch1/3
  Switch1/1 -> Dfc_id/1

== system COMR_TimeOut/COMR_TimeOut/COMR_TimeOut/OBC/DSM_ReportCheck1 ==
  note: Fault report to diagnostic management system
  Dfc_id_nv : Inport  OutDataTypeStr=uint8
  Err : Inport  Port=2
  Heal : Inport  Port=3
  Bit Clear1 : simulink/Logic and Bit Operations/Bit Clear  iBit=4
  Bit Clear2 : simulink/Logic and Bit Operations/Bit Clear  iBit=3
  Bit Set : simulink/Logic and Bit Operations/Bit Set  iBit=4
  Bit Set1 : simulink/Logic and Bit Operations/Bit Set  iBit=3
  Bit Set2 : simulink/Logic and Bit Operations/Bit Set  iBit=3
  Bit Set4 : simulink/Logic and Bit Operations/Bit Set  iBit=7
  Constant1 : Constant  Value=0  OutDataTypeStr=uint8
  Constant7 : Constant  Value=0  OutDataTypeStr=boolean
  Delay2 : Delay  DelayLength=1  InitialCondition=1
  Delay3 : Delay  DelayLength=1  InitialCondition=0
  Logical Operator : Logic  Operator=OR  AllPortsSameDT=off  OutDataTypeStr=boolean
  Switch{1..4} (4 alike) : Switch  Criteria=u2 ~= 0
  Dfc_id : Outport  OutDataTypeStr=uint8
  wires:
  Switch1/1 -> Dfc_id/1
  Constant1/1 -> Switch1/3
  Logical Operator/1 -> Switch1/2
  Heal/1 -> Switch4/2, Logical Operator/1
  Delay3/1 -> Switch4/3
  Bit Clear1/1 -> Bit Set2/1
  Bit Set2/1 -> Switch4/1
  Err/1 -> Switch3/2, Logical Operator/2
  Switch4/1 -> Switch3/3
  Bit Set/1 -> Bit Set1/1
  Bit Set1/1 -> Switch3/1
  Switch2/1 -> Switch1/1, Delay3/1
  Bit Clear2/1 -> Switch2/1
  Switch3/1 -> Switch2/3
  Delay2/1 -> Switch2/2
  Constant7/1 -> Delay2/1
  Bit Set4/1 -> Bit Set/1
  Dfc_id_nv/1 -> Bit Clear1/1, Bit Set4/1, Bit Clear2/1

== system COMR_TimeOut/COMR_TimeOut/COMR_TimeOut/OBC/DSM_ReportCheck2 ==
  note: Fault report to diagnostic management system
  Dfc_id_nv : Inport  OutDataTypeStr=uint8
  Err : Inport  Port=2
  Heal : Inport  Port=3
  Bit Clear1 : simulink/Logic and Bit Operations/Bit Clear  iBit=4
  Bit Clear2 : simulink/Logic and Bit Operations/Bit Clear  iBit=3
  Bit Set : simulink/Logic and Bit Operations/Bit Set  iBit=4
  Bit Set1 : simulink/Logic and Bit Operations/Bit Set  iBit=3
  Bit Set2 : simulink/Logic and Bit Operations/Bit Set  iBit=3
  Bit Set4 : simulink/Logic and Bit Operations/Bit Set  iBit=7
  Constant1 : Constant  Value=0  OutDataTypeStr=uint8
  Constant7 : Constant  Value=0  OutDataTypeStr=boolean
  Delay2 : Delay  DelayLength=1  InitialCondition=1
  Delay3 : Delay  DelayLength=1  InitialCondition=0
  Logical Operator : Logic  Operator=OR  AllPortsSameDT=off  OutDataTypeStr=boolean
  Switch{1..4} (4 alike) : Switch  Criteria=u2 ~= 0
  Dfc_id : Outport  OutDataTypeStr=uint8
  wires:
  Dfc_id_nv/1 -> Bit Clear2/1, Bit Set4/1, Bit Clear1/1
  Bit Set4/1 -> Bit Set/1
  Constant7/1 -> Delay2/1
  Delay2/1 -> Switch2/2
  Switch3/1 -> Switch2/3
  Bit Clear2/1 -> Switch2/1
  Switch2/1 -> Delay3/1, Switch1/1
  Bit Set1/1 -> Switch3/1
  Bit Set/1 -> Bit Set1/1
  Switch4/1 -> Switch3/3
  Err/1 -> Logical Operator/2, Switch3/2
  Bit Set2/1 -> Switch4/1
  Bit Clear1/1 -> Bit Set2/1
  Delay3/1 -> Switch4/3
  Heal/1 -> Logical Operator/1, Switch4/2
  Logical Operator/1 -> Switch1/2
  Constant1/1 -> Switch1/3
  Switch1/1 -> Dfc_id/1

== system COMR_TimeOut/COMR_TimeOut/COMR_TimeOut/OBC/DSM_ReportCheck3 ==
  note: Fault report to diagnostic management system
  Dfc_id_nv : Inport  OutDataTypeStr=uint8
  Err : Inport  Port=2
  Heal : Inport  Port=3
  Bit Clear1 : simulink/Logic and Bit Operations/Bit Clear  iBit=4
  Bit Clear2 : simulink/Logic and Bit Operations/Bit Clear  iBit=3
  Bit Set : simulink/Logic and Bit Operations/Bit Set  iBit=4
  Bit Set1 : simulink/Logic and Bit Operations/Bit Set  iBit=3
  Bit Set2 : simulink/Logic and Bit Operations/Bit Set  iBit=3
  Bit Set4 : simulink/Logic and Bit Operations/Bit Set  iBit=7
  Constant1 : Constant  Value=0  OutDataTypeStr=uint8
  Constant7 : Constant  Value=0  OutDataTypeStr=boolean
  Delay2 : Delay  DelayLength=1  InitialCondition=1
  Delay3 : Delay  DelayLength=1  InitialCondition=0
  Logical Operator : Logic  Operator=OR  AllPortsSameDT=off  OutDataTypeStr=boolean
  Switch{1..4} (4 alike) : Switch  Criteria=u2 ~= 0
  Dfc_id : Outport  OutDataTypeStr=uint8
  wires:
  Switch1/1 -> Dfc_id/1
  Constant1/1 -> Switch1/3
  Logical Operator/1 -> Switch1/2
  Heal/1 -> Switch4/2, Logical Operator/1
  Delay3/1 -> Switch4/3
  Bit Clear1/1 -> Bit Set2/1
  Bit Set2/1 -> Switch4/1
  Err/1 -> Switch3/2, Logical Operator/2
  Switch4/1 -> Switch3/3
  Bit Set/1 -> Bit Set1/1
  Bit Set1/1 -> Switch3/1
  Switch2/1 -> Switch1/1, Delay3/1
  Bit Clear2/1 -> Switch2/1
  Switch3/1 -> Switch2/3
  Delay2/1 -> Switch2/2
  Constant7/1 -> Delay2/1
  Bit Set4/1 -> Bit Set/1
  Dfc_id_nv/1 -> Bit Clear1/1, Bit Set4/1, Bit Clear2/1

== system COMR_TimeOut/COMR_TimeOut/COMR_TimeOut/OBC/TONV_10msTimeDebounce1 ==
  note: Turn On Delay Time Deboune
  u : Inport
  T : Inport  Port=2
  Add : Sum
  Constant1 : Constant  Value=0  OutDataTypeStr=single
  Constant2 : Constant  OutDataTypeStr=uint8
  Constant3 : Constant  Value=0  OutDataTypeStr=uint8
  Constant4 : Constant  Value=0.01  OutDataTypeStr=single
  Delay : Delay  DelayLength=1  InitialCondition=0
  MinMax : MinMax  Inputs=2
  Product : Product  OutMin=[0]  OutMax=[65535]  OutDataTypeStr=single
  Relational Operator : RelationalOperator  Operator=>  OutDataTypeStr=boolean  RndMeth=Simplest
  Switch : Switch  Criteria=u2 ~= 0
  Switch1 : Switch  Criteria=u2 ~= 0
  y : Outport
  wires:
  MinMax/1 -> Add/2
  T/1 -> Relational Operator/2, MinMax/1
  Relational Operator/1 -> y/1
  Delay/1 -> MinMax/2
  Switch/1 -> Add/1
  Product/1 -> Delay/1, Relational Operator/1
  Add/1 -> Product/2
  Constant1/1 -> Switch/3
  Constant4/1 -> Switch/1
  u/1 -> Switch/2, Switch1/2
  Constant2/1 -> Switch1/1
  Constant3/1 -> Switch1/3
  Switch1/1 -> Product/1

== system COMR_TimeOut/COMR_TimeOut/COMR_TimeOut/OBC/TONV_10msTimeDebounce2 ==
  note: Turn On Delay Time Deboune
  u : Inport
  T : Inport  Port=2
  Add : Sum
  Constant1 : Constant  Value=0  OutDataTypeStr=single
  Constant2 : Constant  OutDataTypeStr=uint8
  Constant3 : Constant  Value=0  OutDataTypeStr=uint8
  Constant4 : Constant  Value=0.01  OutDataTypeStr=single
  Delay : Delay  DelayLength=1  InitialCondition=0
  MinMax : MinMax  Inputs=2
  Product : Product  OutMin=[0]  OutMax=[65535]  OutDataTypeStr=single
  Relational Operator : RelationalOperator  Operator=>  OutDataTypeStr=boolean  RndMeth=Simplest
  Switch : Switch  Criteria=u2 ~= 0
  Switch1 : Switch  Criteria=u2 ~= 0
  y : Outport
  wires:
  MinMax/1 -> Add/2
  T/1 -> Relational Operator/2, MinMax/1
  Relational Operator/1 -> y/1
  Delay/1 -> MinMax/2
  Switch/1 -> Add/1
  Product/1 -> Delay/1, Relational Operator/1
  Add/1 -> Product/2
  Constant1/1 -> Switch/3
  Constant4/1 -> Switch/1
  u/1 -> Switch/2, Switch1/2
  Constant2/1 -> Switch1/1
  Constant3/1 -> Switch1/3
  Switch1/1 -> Product/1

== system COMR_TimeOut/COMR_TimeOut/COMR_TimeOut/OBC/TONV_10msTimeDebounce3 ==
  note: Turn On Delay Time Deboune
  u : Inport
  T : Inport  Port=2
  Add : Sum
  Constant1 : Constant  Value=0  OutDataTypeStr=single
  Constant2 : Constant  OutDataTypeStr=uint8
  Constant3 : Constant  Value=0  OutDataTypeStr=uint8
  Constant4 : Constant  Value=0.01  OutDataTypeStr=single
  Delay : Delay  DelayLength=1  InitialCondition=0
  MinMax : MinMax  Inputs=2
  Product : Product  OutMin=[0]  OutMax=[65535]  OutDataTypeStr=single
  Relational Operator : RelationalOperator  Operator=>  OutDataTypeStr=boolean  RndMeth=Simplest
  Switch : Switch  Criteria=u2 ~= 0
  Switch1 : Switch  Criteria=u2 ~= 0
  y : Outport
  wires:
  MinMax/1 -> Add/2
  T/1 -> Relational Operator/2, MinMax/1
  Relational Operator/1 -> y/1
  Delay/1 -> MinMax/2
  Switch/1 -> Add/1
  Product/1 -> Delay/1, Relational Operator/1
  Add/1 -> Product/2
  Constant1/1 -> Switch/3
  Constant4/1 -> Switch/1
  u/1 -> Switch/2, Switch1/2
  Constant2/1 -> Switch1/1
  Constant3/1 -> Switch1/3
  Switch1/1 -> Product/1

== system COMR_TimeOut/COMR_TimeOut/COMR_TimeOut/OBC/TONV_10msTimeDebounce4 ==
  note: Turn On Delay Time Deboune
  u : Inport
  T : Inport  Port=2
  Add : Sum
  Constant1 : Constant  Value=0  OutDataTypeStr=single
  Constant2 : Constant  OutDataTypeStr=uint8
  Constant3 : Constant  Value=0  OutDataTypeStr=uint8
  Constant4 : Constant  Value=0.01  OutDataTypeStr=single
  Delay : Delay  DelayLength=1  InitialCondition=0
  MinMax : MinMax  Inputs=2
  Product : Product  OutMin=[0]  OutMax=[65535]  OutDataTypeStr=single
  Relational Operator : RelationalOperator  Operator=>  OutDataTypeStr=boolean  RndMeth=Simplest
  Switch : Switch  Criteria=u2 ~= 0
  Switch1 : Switch  Criteria=u2 ~= 0
  y : Outport
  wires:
  MinMax/1 -> Add/2
  T/1 -> Relational Operator/2, MinMax/1
  Relational Operator/1 -> y/1
  Delay/1 -> MinMax/2
  Switch/1 -> Add/1
  Product/1 -> Delay/1, Relational Operator/1
  Add/1 -> Product/2
  Constant1/1 -> Switch/3
  Constant4/1 -> Switch/1
  u/1 -> Switch/2, Switch1/2
  Constant2/1 -> Switch1/1
  Constant3/1 -> Switch1/3
  Switch1/1 -> Product/1

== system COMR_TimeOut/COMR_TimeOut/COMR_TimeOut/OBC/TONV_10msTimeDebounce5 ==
  note: Turn On Delay Time Deboune
  u : Inport
  T : Inport  Port=2
  Add : Sum
  Constant1 : Constant  Value=0  OutDataTypeStr=single
  Constant2 : Constant  OutDataTypeStr=uint8
  Constant3 : Constant  Value=0  OutDataTypeStr=uint8
  Constant4 : Constant  Value=0.01  OutDataTypeStr=single
  Delay : Delay  DelayLength=1  InitialCondition=0
  MinMax : MinMax  Inputs=2
  Product : Product  OutMin=[0]  OutMax=[65535]  OutDataTypeStr=single
  Relational Operator : RelationalOperator  Operator=>  OutDataTypeStr=boolean  RndMeth=Simplest
  Switch : Switch  Criteria=u2 ~= 0
  Switch1 : Switch  Criteria=u2 ~= 0
  y : Outport
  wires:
  MinMax/1 -> Add/2
  T/1 -> Relational Operator/2, MinMax/1
  Relational Operator/1 -> y/1
  Delay/1 -> MinMax/2
  Switch/1 -> Add/1
  Product/1 -> Delay/1, Relational Operator/1
  Add/1 -> Product/2
  Constant1/1 -> Switch/3
  Constant4/1 -> Switch/1
  u/1 -> Switch/2, Switch1/2
  Constant2/1 -> Switch1/1
  Constant3/1 -> Switch1/3
  Switch1/1 -> Product/1

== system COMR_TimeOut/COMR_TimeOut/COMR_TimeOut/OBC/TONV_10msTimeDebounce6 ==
  note: Turn On Delay Time Deboune
  u : Inport
  T : Inport  Port=2
  Add : Sum
  Constant1 : Constant  Value=0  OutDataTypeStr=single
  Constant2 : Constant  OutDataTypeStr=uint8
  Constant3 : Constant  Value=0  OutDataTypeStr=uint8
  Constant4 : Constant  Value=0.01  OutDataTypeStr=single
  Delay : Delay  DelayLength=1  InitialCondition=0
  MinMax : MinMax  Inputs=2
  Product : Product  OutMin=[0]  OutMax=[65535]  OutDataTypeStr=single
  Relational Operator : RelationalOperator  Operator=>  OutDataTypeStr=boolean  RndMeth=Simplest
  Switch : Switch  Criteria=u2 ~= 0
  Switch1 : Switch  Criteria=u2 ~= 0
  y : Outport
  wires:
  MinMax/1 -> Add/2
  T/1 -> Relational Operator/2, MinMax/1
  Relational Operator/1 -> y/1
  Delay/1 -> MinMax/2
  Switch/1 -> Add/1
  Product/1 -> Delay/1, Relational Operator/1
  Add/1 -> Product/2
  Constant1/1 -> Switch/3
  Constant4/1 -> Switch/1
  u/1 -> Switch/2, Switch1/2
  Constant2/1 -> Switch1/1
  Constant3/1 -> Switch1/3
  Switch1/1 -> Product/1

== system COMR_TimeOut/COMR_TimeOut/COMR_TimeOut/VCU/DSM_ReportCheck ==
  note: Fault report to diagnostic management system
  Dfc_id_nv : Inport  OutDataTypeStr=uint8
  Err : Inport  Port=2
  Heal : Inport  Port=3
  Bit Clear1 : simulink/Logic and Bit Operations/Bit Clear  iBit=4
  Bit Clear2 : simulink/Logic and Bit Operations/Bit Clear  iBit=3
  Bit Set : simulink/Logic and Bit Operations/Bit Set  iBit=4
  Bit Set1 : simulink/Logic and Bit Operations/Bit Set  iBit=3
  Bit Set2 : simulink/Logic and Bit Operations/Bit Set  iBit=3
  Bit Set4 : simulink/Logic and Bit Operations/Bit Set  iBit=7
  Constant1 : Constant  Value=0  OutDataTypeStr=uint8
  Constant7 : Constant  Value=0  OutDataTypeStr=boolean
  Delay2 : Delay  DelayLength=1  InitialCondition=1
  Delay3 : Delay  DelayLength=1  InitialCondition=0
  Logical Operator : Logic  Operator=OR  AllPortsSameDT=off  OutDataTypeStr=boolean
  Switch{1..4} (4 alike) : Switch  Criteria=u2 ~= 0
  Dfc_id : Outport  OutDataTypeStr=uint8
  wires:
  Dfc_id_nv/1 -> Bit Clear2/1, Bit Set4/1, Bit Clear1/1
  Bit Set4/1 -> Bit Set/1
  Constant7/1 -> Delay2/1
  Delay2/1 -> Switch2/2
  Switch3/1 -> Switch2/3
  Bit Clear2/1 -> Switch2/1
  Switch2/1 -> Delay3/1, Switch1/1
  Bit Set1/1 -> Switch3/1
  Bit Set/1 -> Bit Set1/1
  Switch4/1 -> Switch3/3
  Err/1 -> Logical Operator/2, Switch3/2
  Bit Set2/1 -> Switch4/1
  Bit Clear1/1 -> Bit Set2/1
  Delay3/1 -> Switch4/3
  Heal/1 -> Logical Operator/1, Switch4/2
  Logical Operator/1 -> Switch1/2
  Constant1/1 -> Switch1/3
  Switch1/1 -> Dfc_id/1

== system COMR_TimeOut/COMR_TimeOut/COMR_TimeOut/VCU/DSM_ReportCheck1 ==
  note: Fault report to diagnostic management system
  Dfc_id_nv : Inport  OutDataTypeStr=uint8
  Err : Inport  Port=2
  Heal : Inport  Port=3
  Bit Clear1 : simulink/Logic and Bit Operations/Bit Clear  iBit=4
  Bit Clear2 : simulink/Logic and Bit Operations/Bit Clear  iBit=3
  Bit Set : simulink/Logic and Bit Operations/Bit Set  iBit=4
  Bit Set1 : simulink/Logic and Bit Operations/Bit Set  iBit=3
  Bit Set2 : simulink/Logic and Bit Operations/Bit Set  iBit=3
  Bit Set4 : simulink/Logic and Bit Operations/Bit Set  iBit=7
  Constant1 : Constant  Value=0  OutDataTypeStr=uint8
  Constant7 : Constant  Value=0  OutDataTypeStr=boolean
  Delay2 : Delay  DelayLength=1  InitialCondition=1
  Delay3 : Delay  DelayLength=1  InitialCondition=0
  Logical Operator : Logic  Operator=OR  AllPortsSameDT=off  OutDataTypeStr=boolean
  Switch{1..4} (4 alike) : Switch  Criteria=u2 ~= 0
  Dfc_id : Outport  OutDataTypeStr=uint8
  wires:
  Switch1/1 -> Dfc_id/1
  Constant1/1 -> Switch1/3
  Logical Operator/1 -> Switch1/2
  Heal/1 -> Switch4/2, Logical Operator/1
  Delay3/1 -> Switch4/3
  Bit Clear1/1 -> Bit Set2/1
  Bit Set2/1 -> Switch4/1
  Err/1 -> Switch3/2, Logical Operator/2
  Switch4/1 -> Switch3/3
  Bit Set/1 -> Bit Set1/1
  Bit Set1/1 -> Switch3/1
  Switch2/1 -> Switch1/1, Delay3/1
  Bit Clear2/1 -> Switch2/1
  Switch3/1 -> Switch2/3
  Delay2/1 -> Switch2/2
  Constant7/1 -> Delay2/1
  Bit Set4/1 -> Bit Set/1
  Dfc_id_nv/1 -> Bit Clear1/1, Bit Set4/1, Bit Clear2/1

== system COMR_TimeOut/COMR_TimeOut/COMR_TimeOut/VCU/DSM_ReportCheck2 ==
  note: Fault report to diagnostic management system
  Dfc_id_nv : Inport  OutDataTypeStr=uint8
  Err : Inport  Port=2
  Heal : Inport  Port=3
  Bit Clear1 : simulink/Logic and Bit Operations/Bit Clear  iBit=4
  Bit Clear2 : simulink/Logic and Bit Operations/Bit Clear  iBit=3
  Bit Set : simulink/Logic and Bit Operations/Bit Set  iBit=4
  Bit Set1 : simulink/Logic and Bit Operations/Bit Set  iBit=3
  Bit Set2 : simulink/Logic and Bit Operations/Bit Set  iBit=3
  Bit Set4 : simulink/Logic and Bit Operations/Bit Set  iBit=7
  Constant1 : Constant  Value=0  OutDataTypeStr=uint8
  Constant7 : Constant  Value=0  OutDataTypeStr=boolean
  Delay2 : Delay  DelayLength=1  InitialCondition=1
  Delay3 : Delay  DelayLength=1  InitialCondition=0
  Logical Operator : Logic  Operator=OR  AllPortsSameDT=off  OutDataTypeStr=boolean
  Switch{1..4} (4 alike) : Switch  Criteria=u2 ~= 0
  Dfc_id : Outport  OutDataTypeStr=uint8
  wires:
  Dfc_id_nv/1 -> Bit Clear2/1, Bit Set4/1, Bit Clear1/1
  Bit Set4/1 -> Bit Set/1
  Constant7/1 -> Delay2/1
  Delay2/1 -> Switch2/2
  Switch3/1 -> Switch2/3
  Bit Clear2/1 -> Switch2/1
  Switch2/1 -> Delay3/1, Switch1/1
  Bit Set1/1 -> Switch3/1
  Bit Set/1 -> Bit Set1/1
  Switch4/1 -> Switch3/3
  Err/1 -> Logical Operator/2, Switch3/2
  Bit Set2/1 -> Switch4/1
  Bit Clear1/1 -> Bit Set2/1
  Delay3/1 -> Switch4/3
  Heal/1 -> Logical Operator/1, Switch4/2
  Logical Operator/1 -> Switch1/2
  Constant1/1 -> Switch1/3
  Switch1/1 -> Dfc_id/1

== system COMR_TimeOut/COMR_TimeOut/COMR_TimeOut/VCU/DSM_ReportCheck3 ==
  note: Fault report to diagnostic management system
  Dfc_id_nv : Inport  OutDataTypeStr=uint8
  Err : Inport  Port=2
  Heal : Inport  Port=3
  Bit Clear1 : simulink/Logic and Bit Operations/Bit Clear  iBit=4
  Bit Clear2 : simulink/Logic and Bit Operations/Bit Clear  iBit=3
  Bit Set : simulink/Logic and Bit Operations/Bit Set  iBit=4
  Bit Set1 : simulink/Logic and Bit Operations/Bit Set  iBit=3
  Bit Set2 : simulink/Logic and Bit Operations/Bit Set  iBit=3
  Bit Set4 : simulink/Logic and Bit Operations/Bit Set  iBit=7
  Constant1 : Constant  Value=0  OutDataTypeStr=uint8
  Constant7 : Constant  Value=0  OutDataTypeStr=boolean
  Delay2 : Delay  DelayLength=1  InitialCondition=1
  Delay3 : Delay  DelayLength=1  InitialCondition=0
  Logical Operator : Logic  Operator=OR  AllPortsSameDT=off  OutDataTypeStr=boolean
  Switch{1..4} (4 alike) : Switch  Criteria=u2 ~= 0
  Dfc_id : Outport  OutDataTypeStr=uint8
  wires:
  Switch1/1 -> Dfc_id/1
  Constant1/1 -> Switch1/3
  Logical Operator/1 -> Switch1/2
  Heal/1 -> Switch4/2, Logical Operator/1
  Delay3/1 -> Switch4/3
  Bit Clear1/1 -> Bit Set2/1
  Bit Set2/1 -> Switch4/1
  Err/1 -> Switch3/2, Logical Operator/2
  Switch4/1 -> Switch3/3
  Bit Set/1 -> Bit Set1/1
  Bit Set1/1 -> Switch3/1
  Switch2/1 -> Switch1/1, Delay3/1
  Bit Clear2/1 -> Switch2/1
  Switch3/1 -> Switch2/3
  Delay2/1 -> Switch2/2
  Constant7/1 -> Delay2/1
  Bit Set4/1 -> Bit Set/1
  Dfc_id_nv/1 -> Bit Clear1/1, Bit Set4/1, Bit Clear2/1
